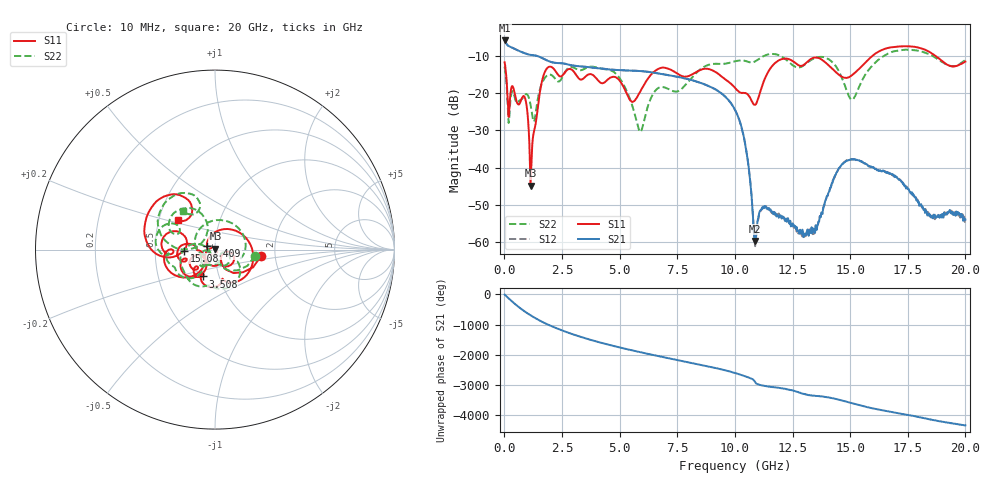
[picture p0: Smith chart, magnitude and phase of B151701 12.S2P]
!  2-Port S-parameters saved by WinCal
! VAR MeasName=S-Parameters (CALIBRATED_DATA) read from VNA (N5244A)
! VAR MeasDate=2015-12-24 19:09:29
! VAR NAME=B151701 12
! VAR FILENAME=B151701 12.S2P
! VAR DATE=2015-12-24 19:09:29
! VAR PHYS_PORTS=1,3
# Hz S DB R 50
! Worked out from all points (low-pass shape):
!   801 points, 10 MHz to 20 GHz, reference 50 ohm
!   highest |S21| = -5.88 dB at 10 MHz (marker M1); lowest = -59.7 dB at 10.85 GHz (marker M2)
!   |S21| within 3 dB of the highest: start of sweep to 708.5 MHz
!   lowest |S11| = -44.8 dB at 1.134 GHz (marker M3), VSWR 1.01, Z = 50.2 + j0.534 ohm
!   |S11| at or under -10 dB: start of sweep to 15.97 GHz; 18.7 GHz to end of sweep
!   |S22| runs from -30.4 to -8.4 dB; largest |S21 - S12| = 0.00087
!   S11 on the Smith chart (normalised r, x): 10 MHz: 1.69, -0.13; 1.409 GHz: 0.91, +0.04; 3.508 GHz: 0.83, -0.26; 15.08 GHz: 0.70, -0.01; 20 GHz: 0.63, +0.22
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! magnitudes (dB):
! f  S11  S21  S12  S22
! 10 MHz  -11.7  -5.9  -5.9  -12.9
! 209.9 MHz  -24.8  -7.5  -7.5  -27.2
! 884.6 MHz  -21.2  -9.3  -9.3  -20.5
! 1.134 GHz  -44.8  -9.7  -9.7  -23.1
! 1.409 GHz  -26.0  -10.0  -10.0  -23.1
! 1.884 GHz  -13.1  -11.3  -11.3  -15.1
! 3.358 GHz  -16.3  -12.8  -12.9  -13.8
! 3.508 GHz  -15.6  -12.9  -12.9  -13.4
! 4.883 GHz  -15.9  -13.8  -13.8  -15.1
! 5.882 GHz  -19.7  -14.1  -14.1  -30.4
! 6.682 GHz  -13.5  -14.7  -14.7  -18.6
! 10.01 GHz  -18.6  -24.5  -24.5  -11.5
! 10.48 GHz  -20.0  -34.9  -34.8  -11.4
! 10.85 GHz  -23.1  -59.7  -59.6  -11.6
! 11.23 GHz  -17.2  -50.4  -50.8  -10.1
! 11.8 GHz  -11.6  -53.1  -52.1  -9.6
! 13.35 GHz  -10.7  -57.7  -56.8  -10.9
! 14.23 GHz  -13.5  -44.2  -43.7  -11.7
! 15.08 GHz  -15.2  -37.7  -37.8  -21.7
! 16.68 GHz  -7.8  -41.4  -41.4  -9.3
! 18.45 GHz  -9.0  -53.1  -52.1  -9.7
! 20 GHz  -11.5  -53.9  -54.2  -11.1
